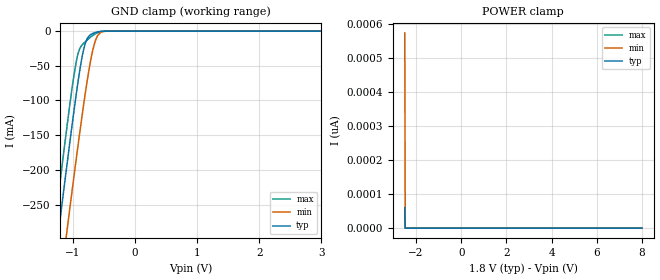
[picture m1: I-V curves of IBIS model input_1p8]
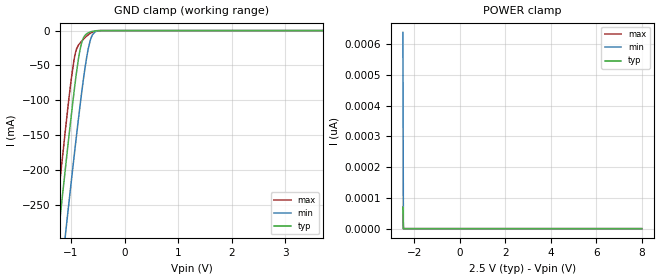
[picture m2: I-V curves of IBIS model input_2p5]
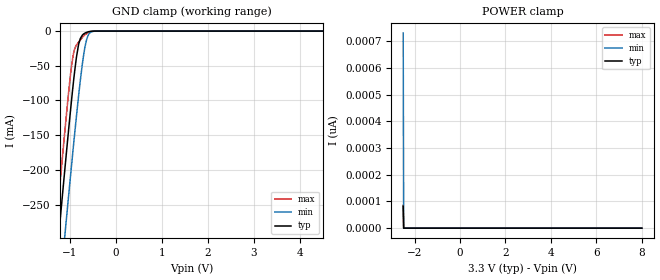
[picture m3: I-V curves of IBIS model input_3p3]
|Texas Instruments Incorporated
| Single Power Supply Single Buffer GATE with 3-State Output CMOS Logic
| Level Shifter
[IBIS Ver]   4.1
[File name]   sn74lv4t125q1.ibs
[File Rev]   1.0
[Date]   2/25/2022
[Source]   Model built from TISPICE simulations at:
   Texas Instruments Incorporated.
   Analog-eLab, HPA
   12500 TI Blvd
   Dallas, TX -75243
   For Support e-mail: elab_ibis@list.ti.com
[Notes]
[Disclaimer]
| This model is designed as an aid for customers of Texas Instruments.
| TI and its licensors and suppliers make no warranties, either expressed
| or implied, with respect to this  model, including the warranties of
| merchantability or fitness for a particular purpose. The model is
| provided solely on an "as is" basis. The entire risk as to its quality
| and performance is with the customer.
[Copyright]
(C) Copyright 2022 Texas Instruments Incorporated.All rights reserved.
|   SN74LV4T125PW
[Component]   SN74LV1T425PW
[Manufacturer]   TI
[Package]   |14 TSSOP  -  PW package
|   typ   min   max
R_pkg   0.19103   0.16967   0.21164
L_pkg   3.05250nH   2.65688nH   3.60685nH
C_pkg   0.48736pF   0.46092pF   0.53275pF
[Pin]  signal_name   model_name   R_pin   L_pin   C_pin
1   1OE   INPUT   0.19696   3.49379nH  0.52991pF
2   1A   INPUT   0.20002   3.01515nH  0.47995pF
3   1Y   OUTPUT   0.17897   2.78188nH  0.46369pF
4   2OE   INPUT   0.16967   2.65688nH  0.46092pF
5   2A   INPUT   0.17977   2.79132nH  0.46440pF
6   2Y   OUTPUT   0.19791   3.00095nH  0.47800pF
7   GND   GND   0.20476   3.55750nH  0.53043pF
8   3Y   OUTPUT   0.19575   3.49014nH  0.52950pF
9   3A   INPUT   0.20186   3.03224nH  0.48111pF
10   3OE   INPUT   0.18274   2.81298nH  0.46552pF
11   4Y   OUTPUT   0.17138   2.66909nH  0.46209pF
12   4A   INPUT   0.18361   2.81712nH  0.46577pF
13   4OE   INPUT   0.19944   3.00908nH  0.47904pF
14   VCC   POWER   0.21164   3.60685nH  0.53275pF
|   Model Selectors
[Model Selector] INPUT
input_1p8   1.8V  digital input
input_2p5   2.5V  digital input
input_3p3   3.3V  digital input
input_5   5.0V  digital input
[Model Selector] OUTPUT
output_1p8   1.8V  digital 3-state
output_2p5   2.5V  digital 3-state
output_3p3   3.3V  digital 3-state
output_5   5.0V  digital 3-state
| Models and submodels in the file (8): input_1p8 (Input), input_2p5 (Input), input_3p3 (Input), input_5 (Input), output_1p8 (3-state), output_2p5 (3-state), output_3p3 (3-state), output_5 (3-state)
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|   input_1p8 Model
[Model]   input_1p8
Model_type   Input
Vinl = 0.5
Vinh = 1
|   typ   min   max
C_comp   3.5pF   3.4pF   3.7pF
[Voltage Range]   1.8   1.65   1.9
[Temperature Range]   25   125   -40
[Power Clamp Reference]   1.8   1.65   1.9
[GND Clamp Reference]   0   0   0
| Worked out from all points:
|   GND clamp passes 1 mA (typ) near -0.59 V on its own axis
[GND Clamp]
|   Voltage   I(typ)   I(min)   I(max)
-2.5V     -1.244A    -1.327A    -1.203A
-1.303V   -342.6mA   -437mA     -288.7mA
-1.23V    -289mA     -383.9mA   -234.5mA
-1.135V   -220.9mA   -316.2mA   -166mA
-1.072V   -176.4mA   -271.7mA   -121.6mA
-998.5mV  -125.8mA   -220.4mA   -72.97mA
-914.5mV  -71.44mA   -163.3mA   -31.85mA
-799mV    -17.49mA   -89.06mA   -15.38mA
-704.5mV  -4.594mA   -38.07mA   -7.858mA
-631mV    -1.797mA   -12.21mA   -3.542mA
-442mV    -17.94uA   -111.5uA   -18.13uA
8V        0A         0A         0A
[POWER Clamp]
|   Voltage   I(typ)   I(min)   I(max)
-2.5V     59.72pA    572.6pA    59.7pA
-2.479V   0A         0A         0A
-2.469V   0A         0A         0A
8V        0A         0A         0A
|   input_2p5 Model
[Model]   input_2p5
Model_type   Input
Vinl = 0.6
Vinh = 1.2
|   typ   min   max
C_comp   3.5pF   3.4pF   3.7pF
[Voltage Range]   2.5   2.3   2.7
[Temperature Range]   25   125   -40
[Power Clamp Reference]   2.5   2.3   2.7
[GND Clamp Reference]   0   0   0
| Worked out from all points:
|   GND clamp passes 1 mA (typ) near -0.59 V on its own axis
[GND Clamp]
|   Voltage   I(typ)   I(min)   I(max)
-2.5V     -1.244A    -1.327A    -1.203A
-1.303V   -342.6mA   -437mA     -288.7mA
-1.23V    -289mA     -383.9mA   -234.5mA
-1.135V   -220.9mA   -316.2mA   -166mA
-1.072V   -176.4mA   -271.7mA   -121.6mA
-998.5mV  -125.8mA   -220.4mA   -72.97mA
-914.5mV  -71.44mA   -163.3mA   -31.85mA
-799mV    -17.49mA   -89.06mA   -15.38mA
-704.5mV  -4.594mA   -38.07mA   -7.858mA
-631mV    -1.797mA   -12.21mA   -3.542mA
-442mV    -17.94uA   -111.5uA   -18.13uA
8V        0A         0A         0A
[POWER Clamp]
|   Voltage   I(typ)   I(min)   I(max)
-2.5V     69.8pA     637.9pA    71.28pA
-2.479V   0A         0A         0A
-2.469V   0A         0A         0A
8V        0A         0A         0A
|   input_3p3 Model
[Model]   input_3p3
Model_type   Input
Vinl = 0.75
Vinh = 1.35
|   typ   min   max
C_comp   3.5pF   3.4pF   3.7pF
[Voltage Range]   3.3   3   3.6
[Temperature Range]   25   125   -40
[Power Clamp Reference]   3.3   3   3.6
[GND Clamp Reference]   0   0   0
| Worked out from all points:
|   GND clamp passes 1 mA (typ) near -0.59 V on its own axis
[GND Clamp]
|   Voltage   I(typ)   I(min)   I(max)
-2.5V     -1.244A    -1.327A    -1.203A
-1.313V   -350.3mA   -444.6mA   -296.5mA
-1.23V    -289mA     -383.9mA   -234.5mA
-1.125V   -213.4mA   -308.8mA   -158.5mA
-1.072V   -176.4mA   -271.7mA   -121.6mA
-977.5mV  -111.7mA   -206mA     -60.6mA
-914.5mV  -71.44mA   -163.3mA   -31.85mA
-799mV    -17.49mA   -89.06mA   -15.38mA
-704.5mV  -4.594mA   -38.07mA   -7.858mA
-631mV    -1.797mA   -12.21mA   -3.542mA
-442mV    -17.94uA   -111.5uA   -18.13uA
8V        0A         0A         0A
[POWER Clamp]
|   Voltage   I(typ)   I(min)   I(max)
-2.5V     82.15pA    731.9pA    85.63pA
-2.479V   0A         0A         0A
-1mV      0A         0A         0A
8V        0A         0A         0A
